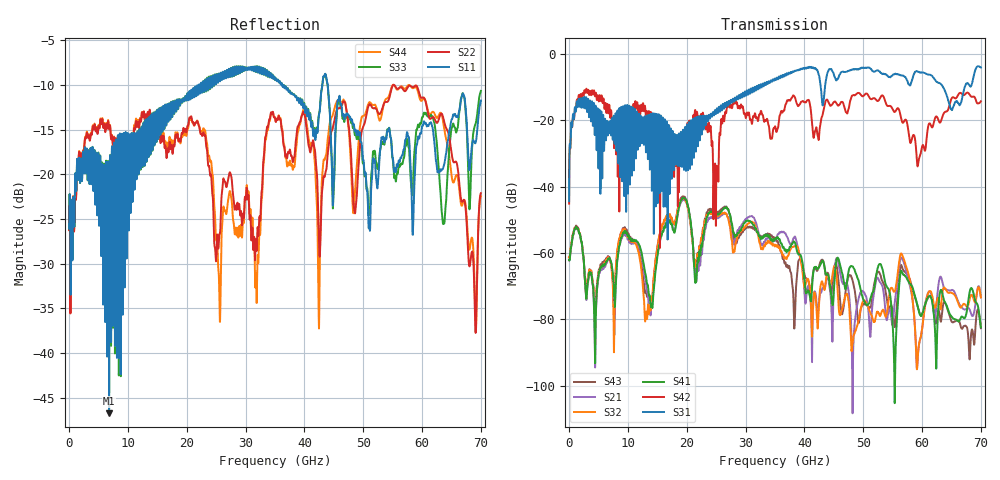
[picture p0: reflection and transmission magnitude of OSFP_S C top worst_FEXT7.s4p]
! AWR Design Environment (8415) Mon Jan 07 17:21:30 2019
! Document = 'OSFP Channel_S'
! nPorts: 4, nXvals: 7001
# HZ S DB R 50
!Freq DBS11 AngS11 DBS12 AngS12 DBS13 AngS13 DBS14 AngS14
!	DBS21 AngS21 DBS22 AngS22 DBS23 AngS23 DBS24 AngS24
!	DBS31 AngS31 DBS32 AngS32 DBS33 AngS33 DBS34 AngS34
!	DBS41 AngS41 DBS42 AngS42 DBS43 AngS43 DBS44 AngS44
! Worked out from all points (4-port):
!   7000 points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, 10 MHz to 70 GHz, reference 50 ohm
!   strongest paths, dB at 10 MHz, 17.51 GHz, 35.01 GHz, 52.51 GHz, 70 GHz:
!     S31: -44.4, -26.6, -7.4, -4.9, -4.0
!     S42: -45.1, -32.2, -21.8, -14.1, -14.3
!     S41: -62.1, -51.8, -55.8, -64.2, -82.4
!     S32: -61.3, -49.8, -57.8, -77.9, -73.3
!     S21: -62.2, -51.4, -56.1, -67.5, -73.3
!     S43: -61.3, -49.9, -55.9, -65.7, -82.6
!   lowest |S11| = -46.8 dB at 6.81 GHz (marker M1), VSWR 1.01, Z = 50.2 + j0.399 ohm
!   |S11| at or under -10 dB: start of sweep to 22.11 GHz; 36.23 GHz to 43.05 GHz (6.816 GHz wide, 17.2 % of centre); 43.96 GHz to end of sweep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
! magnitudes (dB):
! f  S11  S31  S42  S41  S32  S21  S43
! 10 MHz  -26.1  -44.4  -45.1  -62.1  -61.3  -62.2  -61.3
! 6.81 GHz  -46.8  -22.7  -15.4  -61.5  -61.5  -61.9  -61.2
! 13.23 GHz  -16.4  -18.5  -17.2  -69.1  -79.7  -71.7  -73.1
! 19.42 GHz  -11.5  -23.5  -26.2  -43.4  -43.5  -43.9  -42.9
! 21.51 GHz  -10.3  -25.3  -17.6  -68.8  -62.7  -66.7  -63.8
! 26.67 GHz  -9.3  -15.9  -17.9  -46.2  -48.1  -48.1  -46.0
! 70 GHz  -11.8  -4.0  -14.3  -82.4  -73.3  -73.3  -82.6
